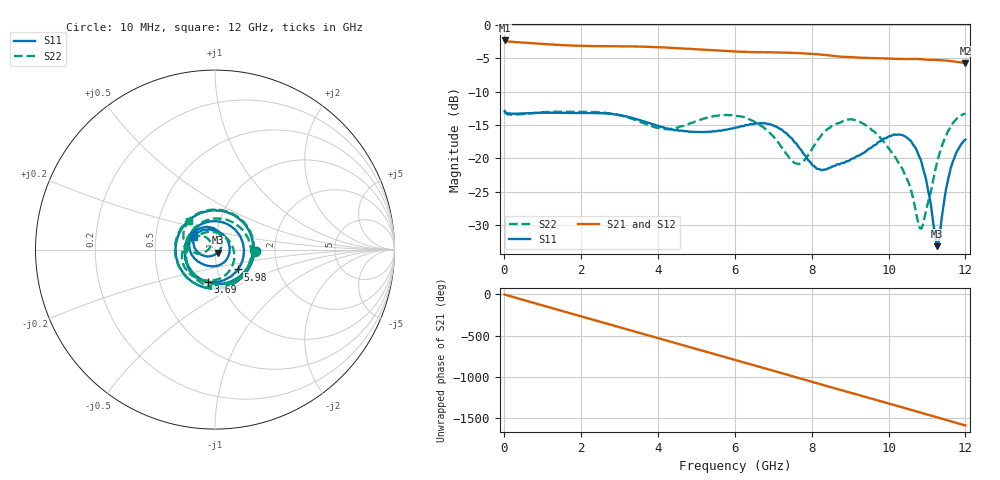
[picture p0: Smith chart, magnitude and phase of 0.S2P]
!Agilent Technologies,E5071C,MY46316741,A.11.02
!Date: Fri Apr 15 15:47:38 2022
!Data & Calibration Information:
!Freq	S11:SOLT2(ON)	S21:SOLT2(ON)	S12:SOLT2(ON)	S22:SOLT2(ON)
!PortZ  Port1:50+j0  Port2:50+j0
!Above PortZ is port z conversion or system Z0 setting when saving the data.
!When reading, reference impedance value at option line is always used.
# Hz S dB R 50
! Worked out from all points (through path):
!   1200 points, 10 MHz to 12 GHz, reference 50 ohm
!   highest |S21| = -2.34 dB at 10 MHz (marker M1); lowest = -5.7 dB at 12 GHz (marker M2)
!   group delay of S21, straight-line fit = 366 ps
!   lowest |S11| = -33.1 dB at 11.27 GHz (marker M3), VSWR 1.05, Z = 51.4 - j1.72 ohm
!   |S11| at or under -10 dB: start of sweep to end of sweep
!   |S22| runs from -30.5 to -13.0 dB; largest |S21 - S12| = 0.0043
!   S11 on the Smith chart (normalised r, x): 10 MHz: 1.58, -0.04; 3.69 GHz: 0.86, -0.33; 5.98 GHz: 1.26, -0.29; 12 GHz: 0.78, +0.11
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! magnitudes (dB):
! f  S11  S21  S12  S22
! 10 MHz  -12.9  -2.3  -2.3  -13.0
! 2.01 GHz  -13.2  -3.1  -3.1  -13.0
! 3.69 GHz  -14.6  -3.3  -3.3  -14.9
! 4.01 GHz  -15.1  -3.3  -3.3  -15.5
! 4.96 GHz  -16.0  -3.7  -3.6  -14.5
! 5.98 GHz  -15.5  -4.0  -4.0  -13.6
! 6.01 GHz  -15.4  -4.0  -4.0  -13.6
! 6.89 GHz  -14.9  -4.1  -4.1  -16.0
! 7.58 GHz  -17.7  -4.2  -4.2  -20.7
! 8.01 GHz  -20.9  -4.3  -4.3  -18.6
! 8.44 GHz  -21.5  -4.6  -4.6  -15.5
! 9.01 GHz  -20.2  -4.9  -4.8  -14.2
! 9.48 GHz  -18.6  -4.9  -5.0  -15.3
! 10.01 GHz  -16.7  -5.1  -5.1  -18.5
! 10.49 GHz  -16.9  -5.1  -5.1  -23.2
! 10.84 GHz  -20.2  -5.1  -5.1  -30.5
! 11.01 GHz  -24.2  -5.2  -5.2  -27.0
! 11.21 GHz  -31.5  -5.2  -5.2  -21.9
! 11.27 GHz  -33.1  -5.3  -5.3  -20.4
! 11.62 GHz  -21.4  -5.4  -5.4  -15.2
! 11.79 GHz  -18.9  -5.6  -5.6  -14.0
! 12 GHz  -17.2  -5.7  -5.7  -13.3
